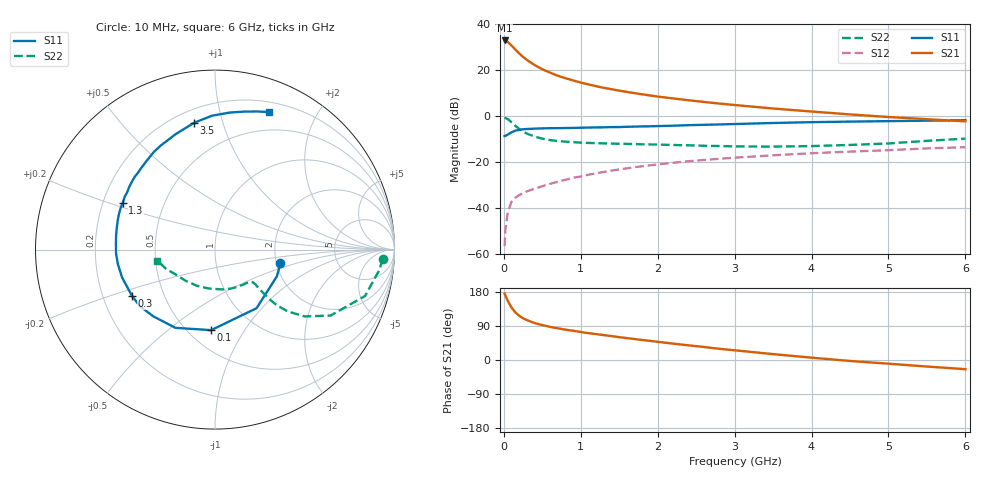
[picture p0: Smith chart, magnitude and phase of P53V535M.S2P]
! SIEMENS Small Signal Semiconductors
! BFP183
! Si NPN RF Bipolar Junction Transistor in SOT143
! VCE = 3.5 V  IC = 35 mA
! Common Emitter S-Parameters:  March  1996
# GHz  S  MA  R  50
!  f  S11  S21  S12  S22
! GHz  MAG  ANG  MAG  ANG  MAG  ANG  MAG  ANG
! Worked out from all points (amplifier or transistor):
!   36 points, 10 MHz to 6 GHz, reference 50 ohm
!   highest |S21| = 33.0 dB at 10 MHz (marker M1)
!   |S21| within 3 dB of that: start of sweep to 122.2 MHz
!   unconditionally stable (mu >= 1): 563.5 MHz to 5.634 GHz
!   at 250 MHz: K = 0.65, MSG = 29.6 dB, |S12| = -33.4 dB
!   at 1.4 GHz: K = 1.19, MAG = 15.1 dB, |S12| = -23.6 dB
!   at 6 GHz: K = 0.96, MSG = 5.6 dB, |S12| = -13.4 dB
!   S11 on the Smith chart (normalised r, x): 10 MHz: 2.10, -0.37; 100 MHz: 0.64, -0.72; 300 MHz: 0.33, -0.23; 1.3 GHz: 0.28, +0.22; 3.5 GHz: 0.28, +0.81; 6 GHz: 0.30, +1.43
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0.01  0.3727 -11.8  44.69 175.0  0.0015 80.4  0.9353 -3.2
0.02  0.3756 -23.4  44.36 170.5  0.0034 85.9  0.9232 -7.0
0.05  0.4003 -54.7  41.77 156.5  0.008 75.3  0.8747 -17.2
0.1  0.4491 -92.7  34.58 138.4  0.0139 60.1  0.7417 -29.7
0.15  0.4884 -116.8  28.29 125.6  0.017 54.6  0.6228 -36.7
0.2  0.5064 -132.7  23.35 116.6  0.0194 51.8  0.533 -40.3
0.25  0.5239 -143.0  19.6 110.0  0.0213 51.3  0.4686 -41.9
0.3  0.5296 -150.8  16.88 105.3  0.0233 51.9  0.4207 -42.3
0.4  0.5406 -163.3  13.06 97.5  0.0268 53.6  0.3619 -42.0
0.5  0.547 -171.4  10.56 92.1  0.0302 54.3  0.3268 -41.5
0.6  0.5518 -177.8  8.942 87.5  0.034 55.9  0.3049 -40.9
0.7  0.5529 176.6  7.643 83.6  0.0378 57.3  0.2906 -40.6
0.8  0.5566 171.9  6.76 80.1  0.0416 58.2  0.281 -40.8
1.1  0.5704 159.8  4.946 70.9  0.0538 58.7  0.2637 -43.0
1.3  0.5765 153.2  4.162 65.6  0.0618 58.0  0.2581 -45.6
1.7  0.598 140.7  3.19 55.3  0.0781 56.0  0.2495 -52.3
2.2  0.6255 127.1  2.45 43.2  0.0976 51.8  0.2379 -62.9
2.8  0.6656 112.8  1.898 29.6  0.1191 46.1  0.2262 -78.7
3.5  0.7164 99.3  1.48 15.5  0.142 39.5  0.2195 -100.2
4.5  0.7678 83.9  1.101 -2.6  0.1708 30.0  0.2386 -133.3
5.5  0.8048 73.0  0.867 -17.3  0.2007 21.9  0.293 -158.5
6  0.8241 68.4  0.778 -24.2  0.2131 17.1  0.3275 -169.3
